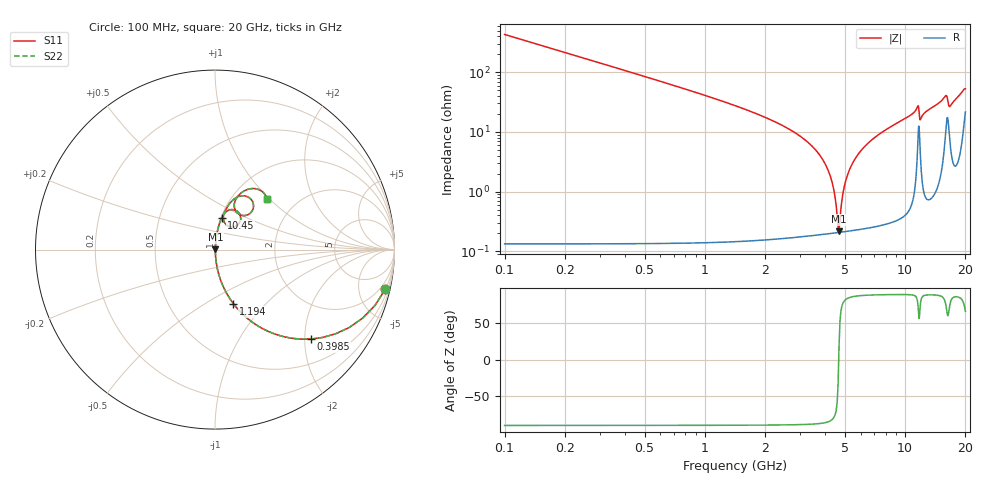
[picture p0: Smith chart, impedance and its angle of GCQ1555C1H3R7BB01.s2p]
!Murata Part Number: GCQ1555C1H3R7BB01
!These Parameters are Measured in Series Mode Connection
!Data Generated on Jan 08, 2026
!  o--ll--o
!Port1  Port2
!  o------o
!Operation Temp=25[degC], DC Bias Voltage=0[V]
!Freq. Start=100[MHz] Stop=20[GHz] 401[Steps]
# Hz S RI R 50
!Freq.(Hz) S11(Real) S11(Imag) S21(Real) S21(Imag) S12(Real) S12(Imag) S22(Real) S22(Imag)
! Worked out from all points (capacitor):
!   401 points, 100 MHz to 20 GHz, reference 50 ohm
!   read as one part in series: C = 3.7 pF near 199.5 MHz
!   lowest |Z| = 216 mohm at 4.677 GHz (marker M1)
!   series resonance near 4.661 GHz, so ESL is about 320 pH
!   S11 on the Smith chart (normalised r, x): 100 MHz: 1.00, -8.60; 398.5 MHz: 1.00, -2.14; 1.194 GHz: 1.00, -0.67; 10.45 GHz: 1.01, +0.37; 20 GHz: 1.43, +0.96
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1e8  0.9486 -0.2206  0.0514 0.2206  0.0514 0.2206  0.9486 -0.2206
3.985e8  0.5345 -0.4982  0.4655 0.4982  0.4655 0.4982  0.5345 -0.4982
7.4675e8  0.2401 -0.4259  0.7599 0.4259  0.7599 0.4259  0.2401 -0.4259
1.1945e9  0.1028 -0.3015  0.8972 0.3015  0.8972 0.3015  0.1028 -0.3015
3.43325e9  0.00511 -0.0571  0.9949 0.0571  0.9949 0.0571  0.00511 -0.0571
4.1795e9  0.00238 -0.0202  0.9976 0.0202  0.9976 0.0202  0.00238 -0.0202
4.42825e9  0.00211 -0.0095  0.9979 0.0095  0.9979 0.0095  0.00211 -0.0095
4.5775e9  0.00206 -0.00336  0.9979 0.00336  0.9979 0.00336  0.00206 -0.00336
4.677e9  0.00207 0.000624  0.9979 -0.000624  0.9979 -0.000624  0.00207 0.000624
4.9755e9  0.00227 0.0121  0.9977 -0.0121  0.9977 -0.0121  0.00227 0.0121
5.32375e9  0.0028 0.0248  0.9972 -0.0248  0.9972 -0.0248  0.0028 0.0248
5.92075e9  0.00434 0.045  0.9957 -0.045  0.9957 -0.045  0.00434 0.045
6.7665e9  0.00761 0.0713  0.9924 -0.0713  0.9924 -0.0713  0.00761 0.0713
1.005e10  0.0316 0.1635  0.9684 -0.1635  0.9684 -0.1635  0.0316 0.1635
1.0448e10  0.0368 0.1757  0.9632 -0.1757  0.9632 -0.1757  0.0368 0.1757
1.15425e10  0.1048 0.2222  0.8952 -0.2222  0.8952 -0.2222  0.1048 0.2222
1.19405e10  0.057 0.1443  0.943 -0.1443  0.943 -0.1443  0.057 0.1443
1.338325e10  0.0634 0.229  0.9366 -0.229  0.9366 -0.229  0.0634 0.229
1.59205e10  0.1895 0.2899  0.8105 -0.2899  0.8105 -0.2899  0.1895 0.2899
1.67165e10  0.1186 0.2109  0.8814 -0.2109  0.8814 -0.2109  0.1186 0.2109
1.89055e10  0.1833 0.3358  0.8167 -0.3358  0.8167 -0.3358  0.1833 0.3358
2e10  0.289 0.2816  0.711 -0.2816  0.711 -0.2816  0.289 0.2816
